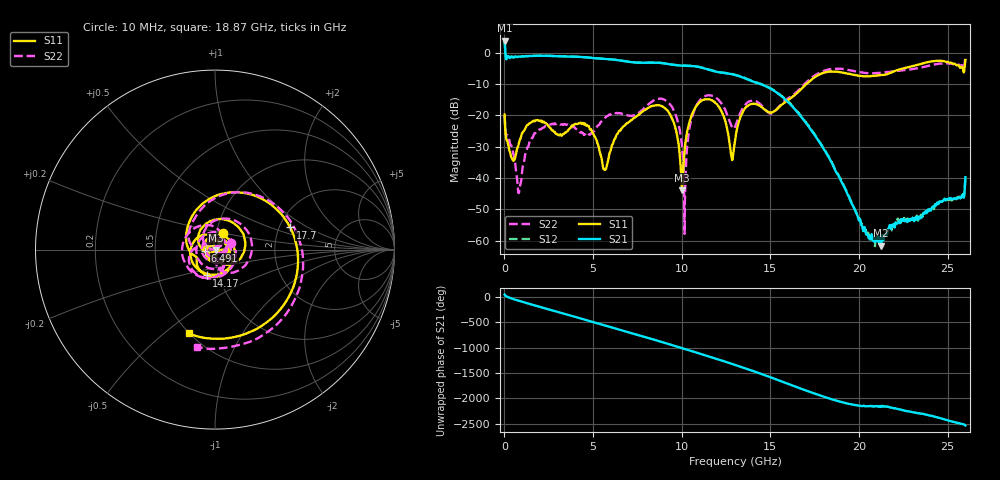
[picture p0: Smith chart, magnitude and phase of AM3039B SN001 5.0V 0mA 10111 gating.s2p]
!Agilent Technologies,E8364B,MY43040894,A.07.50.67
!Agilent E8364B: A.07.50.67
!Date: Tuesday, June 28, 2016 08:09:37
!Correction: S11(Full 2 Port(1,2))
!S21(Full 2 Port(1,2))
!S12(Full 2 Port(1,2))
!S22(Full 2 Port(1,2))
!S2P File: Measurements: S11, S21, S12, S22:
# Hz S  dB  R 50
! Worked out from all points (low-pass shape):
!   1601 points, 10 MHz to 26 GHz, reference 50 ohm
!   highest |S21| = 3.80 dB at 10 MHz (marker M1); lowest = -61.6 dB at 21.26 GHz (marker M2)
!   |S21| within 3 dB of the highest: start of sweep to 43.89 MHz
!   lowest |S11| = -44.0 dB at 10.02 GHz (marker M3), VSWR 1.01, Z = 50.5 - j0.412 ohm
!   |S11| at or under -10 dB: start of sweep to 17.04 GHz
!   |S22| runs from -57.8 to -1.3 dB; largest |S21 - S12| = 0.024
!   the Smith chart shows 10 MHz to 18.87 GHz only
!   S11 on the Smith chart (normalised r, x): 10 MHz: 1.08, +0.20; 6.491 GHz: 0.89, -0.01; 14.17 GHz: 0.87, -0.26; 17.7 GHz: 2.30, +0.70; 18.87 GHz: 0.50, -0.61
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1e7  -19.80 63.0  3.80 41.1  3.85 41.9  -20.30 23.4
7.572125e8  -30.07 99.9  -1.35 -75.1  -1.30 -74.9  -43.17 -117.5
1.731838e9  -21.86 10.5  -1.07 -174.4  -1.03 -174.2  -25.78 -17.0
2.787681e9  -25.20 -142.6  -1.14 81.0  -1.07 81.0  -22.84 -177.2
3.583625e9  -24.89 57.6  -1.28 2.7  -1.22 2.7  -23.06 51.9
4.347081e9  -22.70 -65.0  -1.43 -73.8  -1.40 -73.7  -25.43 -82.4
5.402925e9  -32.10 126.4  -1.93 -179.7  -1.90 -179.5  -22.39 42.1
6.491256e9  -24.94 -172.7  -2.50 69.8  -2.43 70.0  -19.36 -140.5
7.368419e9  -20.66 48.8  -3.18 -17.3  -3.14 -17.2  -19.93 57.3
8.684162e9  -16.77 -142.4  -3.28 -151.3  -3.21 -151.0  -14.80 -156.3
1.001615e10  -43.97 -40.1  -4.16 69.4  -4.10 69.7  -29.75 29.1
1.139687e10  -14.89 50.1  -5.25 -82.9  -5.19 -82.7  -13.72 34.3
1.3005e10  -28.04 -0.1  -7.13 98.5  -7.04 98.9  -23.63 -61.8
1.417455e10  -16.41 -108.1  -9.54 -39.8  -9.45 -39.3  -15.49 -142.5
1.734208e10  -8.53 52.9  -25.02 -85.8  -24.79 -85.6  -7.95 44.4
1.769944e10  -7.19 16.4  -27.99 -129.1  -27.77 -128.8  -6.66 11.1
1.886899e10  -6.20 -107.5  -39.62 103.5  -39.29 102.2  -5.17 -100.4
2.125682e10  -7.14 57.6  -61.62 6.2  -59.78 0.7  -6.48 68.5
2.167916e10  -6.68 29.4  -55.98 -6.1  -56.07 -15.7  -6.19 37.4
2.328729e10  -3.93 -92.9  -52.26 -127.2  -52.56 -138.1  -5.04 -81.4
2.440811e10  -2.64 175.6  -47.87 149.3  -48.19 148.1  -3.64 -167.5
2.6e10  -2.36 -8.1  -39.75 -11.2  -39.54 -12.3  -1.29 25.7
